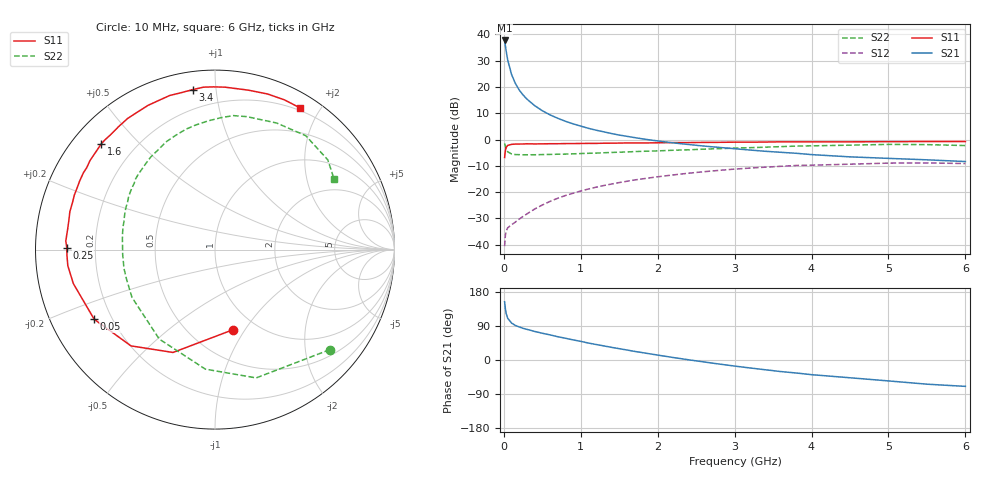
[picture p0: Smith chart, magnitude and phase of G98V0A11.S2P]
! SIEMENS Small Signal Semiconductors
! BFG235
! Si NPN RF Bipolar Junction Transistor in SOT223
! VCE = 8 V  IC = 110 mA
! Common Emitter S-Parameters:  July  1994
# GHz  S  MA  R  50
!  f  S11  S21  S12  S22
! GHz  MAG  ANG  MAG  ANG  MAG  ANG  MAG  ANG
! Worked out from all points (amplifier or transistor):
!   40 points, 10 MHz to 6 GHz, reference 50 ohm
!   highest |S21| = 37.7 dB at 10 MHz (marker M1)
!   |S21| within 3 dB of that: start of sweep to 25.19 MHz
!   unconditionally stable (mu >= 1): 462 MHz to 1.421 GHz
!   at 200 MHz: K = 0.77, MSG = 24.6 dB, |S12| = -30.3 dB
!   at 1.5 GHz: K = 0.99, MSG = 9.0 dB, |S12| = -16.3 dB
!   at 6 GHz: K = 0.89, MSG = 0.4 dB, |S12| = -9.1 dB
!   S11 on the Smith chart (normalised r, x): 10 MHz: 0.79, -0.89; 50 MHz: 0.13, -0.26; 250 MHz: 0.10, +0.01; 1.6 GHz: 0.08, +0.39; 3.4 GHz: 0.09, +0.87; 6 GHz: 0.17, +1.76
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0.01  0.4574 -77.2  77.03 153.6  0.0094 65.1  0.8483 -41.1
0.02  0.619 -112.2  61.4 135.1  0.0151 50.3  0.7508 -72.2
0.03  0.7119 -131.1  48.85 123.1  0.0181 41.6  0.6682 -94.6
0.05  0.777 -150.0  32.82 110.2  0.021 33.7  0.5873 -121.9
0.1  0.8116 -166.5  17.43 97.5  0.024 35.1  0.5337 -150.1
0.15  0.8248 -173.7  11.73 91.2  0.027 40.5  0.5195 -162.1
0.2  0.8254 -177.4  8.783 87.2  0.0307 44.4  0.5177 -168.7
0.25  0.826 179.2  7.075 83.6  0.0346 48.6  0.5148 -173.2
0.3  0.8327 176.7  5.906 80.9  0.0386 51.0  0.5151 -177.0
0.4  0.8287 172.1  4.443 75.4  0.0478 54.6  0.5155 177.8
0.5  0.8307 168.3  3.549 70.6  0.057 56.2  0.5193 173.5
0.6  0.8359 165.3  2.962 66.3  0.0668 56.7  0.5232 169.7
0.7  0.8363 161.6  2.551 61.5  0.0767 56.7  0.5277 166.3
0.9  0.8414 156.0  1.997 53.1  0.0956 54.2  0.5367 160.2
1.1  0.849 149.7  1.639 44.7  0.115 51.3  0.5497 154.2
1.6  0.8652 137.2  1.156 26.4  0.1613 41.8  0.582 140.7
2.2  0.878 123.7  0.868 6.6  0.213 29.1  0.6278 124.8
3.2  0.8943 102.2  0.634 -21.0  0.2876 6.0  0.7028 98.7
3.4  0.8999 97.9  0.6 -25.8  0.2993 1.2  0.7183 93.0
4.5  0.9076 78.2  0.47 -46.9  0.3412 -24.1  0.7846 64.0
5.5  0.9196 65.1  0.413 -63.8  0.3608 -46.2  0.803 38.5
6  0.9208 59.0  0.383 -69.6  0.3504 -54.7  0.7714 30.7
